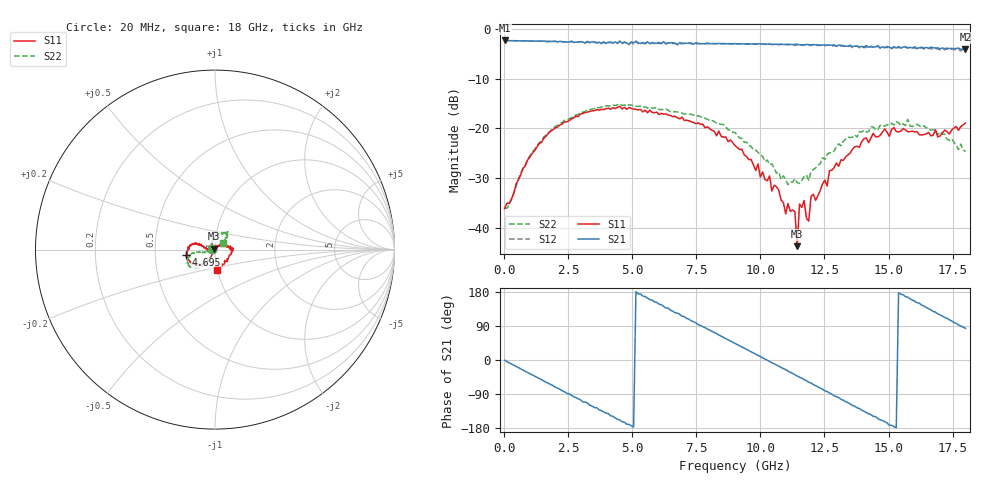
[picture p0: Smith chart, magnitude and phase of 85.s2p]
!Agilent Technologies,N5230A,US43500223,A.07.50.48
!Agilent N5230A: A.07.50.48
!Date: Saturday, January 16, 2016 14:26:48
!Correction: S11(Full 2 Port(1,2))
!S21(Full 2 Port(1,2))
!S12(Full 2 Port(1,2))
!S22(Full 2 Port(1,2))
!S2P File: Measurements: S11, S21, S12, S22:
# Hz S  dB  R 50
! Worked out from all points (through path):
!   201 points, 20 MHz to 18 GHz, reference 50 ohm
!   highest |S21| = -2.31 dB at 20 MHz (marker M1); lowest = -4.1 dB at 18 GHz (marker M2)
!   group delay of S21, straight-line fit = 98 ps
!   lowest |S11| = -43.7 dB at 11.44 GHz (marker M3), VSWR 1.01, Z = 49.6 + j0.482 ohm
!   |S11| at or under -10 dB: start of sweep to end of sweep
!   |S22| runs from -36.1 to -15.1 dB; largest |S21 - S12| = 0.064
!   S11 on the Smith chart (normalised r, x): 20 MHz: 0.97, +0.00; 4.695 GHz: 0.72, -0.05; 18 GHz: 1.00, -0.23
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2e7  -36.14 176.7  -2.31 -0.7  -2.32 -0.8  -35.99 175.5
1.5483e9  -22.00 -125.2  -2.41 -55.3  -2.43 -55.8  -21.75 -119.5
3.0766e9  -16.95 -144.8  -2.63 -110.8  -2.62 -110.5  -16.74 -136.5
4.6948e9  -15.78 -168.6  -2.70 -163.9  -2.61 -165.5  -15.30 -150.9
6.0433e9  -17.22 171.0  -2.74 147.4  -2.89 145.0  -16.23 -161.1
7.4817e9  -19.08 162.0  -2.76 98.0  -2.97 95.4  -17.55 -168.5
9.01e9  -23.45 163.2  -2.95 43.9  -3.01 41.4  -20.82 -169.7
1.00888e10  -28.75 168.7  -3.05 5.6  -3.05 3.2  -25.65 -164.7
1.07181e10  -32.46 175.9  -3.10 -16.4  -3.17 -19.4  -28.82 -173.0
1.09878e10  -37.20 163.1  -3.08 -25.5  -3.17 -29.3  -30.29 -179.0
1.13474e10  -36.81 133.6  -3.10 -38.5  -3.28 -42.0  -30.14 159.2
1.14373e10  -43.71 131.8  -3.07 -42.2  -3.20 -44.5  -30.91 155.7
1.15272e10  -35.24 131.8  -3.18 -45.5  -3.15 -48.7  -31.09 148.5
1.1707e10  -34.52 80.5  -3.17 -51.7  -3.20 -54.4  -29.71 134.3
1.18868e10  -38.68 103.5  -3.15 -58.4  -3.31 -61.2  -30.46 135.0
1.19767e10  -33.69 87.0  -3.20 -60.9  -3.29 -63.6  -28.62 124.0
1.20666e10  -33.25 65.6  -3.14 -64.6  -3.16 -67.8  -28.29 114.6
1.3505e10  -24.97 19.0  -3.27 -116.0  -3.37 -119.7  -21.86 80.4
1.4404e10  -21.01 12.3  -3.66 -148.8  -3.65 -152.2  -19.75 66.9
1.50333e10  -21.61 2.8  -3.64 -172.3  -3.93 -174.4  -19.30 62.0
1.65616e10  -20.81 -37.0  -3.91 135.6  -3.92 130.3  -19.94 48.3
1.8e10  -18.93 -83.0  -4.10 83.6  -4.24 77.8  -24.67 38.0
